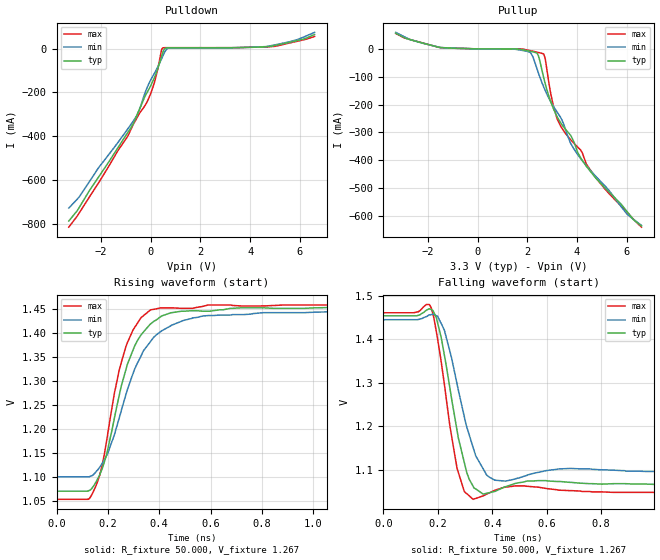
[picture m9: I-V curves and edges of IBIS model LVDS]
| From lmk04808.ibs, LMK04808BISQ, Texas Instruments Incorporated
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|   Model LVDS
[Model]   LVDS
Model_type   Output
Polarity   Non-Inverting
Vmeas = 1.25
Vref = 1.25
Cref = 0pF
Rref = 50
|   typ   min   max
|   (nom PVT)   (slow PVT)   (fast PVT)
C_comp   1.2694p   1.2464p   1.3920p
|C_comp (High state)   1.2694p   1.2464p   1.3920p
|C_comp (Low state)   1.7368p   1.7367p   1.7369p
[Voltage Range]   3.3   3.135   3.465
[Temperature Range]   45   125   -40
[Pullup Reference]   3.3   3.135   3.465
[Pulldown Reference]   0   0   0
[Power Clamp Reference]   3.3   3.135   3.465
[GND Clamp Reference]   0   0   0
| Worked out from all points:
|   slope of the pulldown table from 0 to 0.495 V, typ, clamps not added: 3.2 ohm
|   slope of the pullup table from 0 to 0.495 V, typ, clamps not added: 2.77 kohm
|   falling waveform, R_fixture 50.000, V_fixture 1.267: 20-80 % time 65.4ps typ, 78ps min, 57.7ps max; typ from 1.45 V to 1.07 V
|   rising waveform, R_fixture 50.000, V_fixture 1.267: 20-80 % time 113ps typ, 145ps min, 93.3ps max; typ from 1.07 V to 1.45 V
[Pulldown]
|   Voltage   I(typ)   I(min)   I(max)
-3.3V     -787.7mA   -728.5mA   -815.8mA
-2.869V   -723.8mA   -675.6mA   -748.8mA
-2.087V   -584.3mA   -542.1mA   -610.8mA
-686.4mV  -339.2mA   -328.2mA   -342.8mA
-468.6mV  -280.5mA   -281.5mA   -298.2mA
-181.5mV  -206.8mA   -187.5mA   -250.5mA
145.2mV   -132.5mA   -113mA     -154.9mA
476.8mV   -19.91mA   -35.88mA   2.577mA
561mV     564.3uA    -15.24mA   4.215mA
699.6mV   3.868mA    2.101mA    4.258mA
4.635V    8.376mA    9.221mA    7.753mA
6.595V    64.54mA    74.45mA    55.51mA
[Pullup]
|   Voltage   I(typ)   I(min)   I(max)
-3.3V     56.64mA    59.79mA    55.64mA
-1.488V   4.87mA     5.063mA    4.727mA
2.086V    -8.017mA   -10.91mA   -5.469mA
2.442V    -23.36mA   -85.47mA   -12.67mA
2.655V    -101.9mA   -135.9mA   -18.19mA
3.056V    -215.8mA   -207.2mA   -207mA
3.333V    -264.3mA   -245.2mA   -276.1mA
3.739V    -310mA     -338.7mA   -326.1mA
4.125V    -388.1mA   -391.9mA   -361.5mA
4.783V    -466.9mA   -460.8mA   -466.5mA
6.021V    -585.4mA   -594.9mA   -587.7mA
6.595V    -636.8mA   -634.7mA   -640.9mA
[Ramp]
R_load = 50
|   typ   min   max
dV/dt_r   0.231387/1.13087e-10   0.206921/1.44841e-10   0.243676/9.35061e-11
dV/dt_f   0.233919/6.51324e-11   0.206921/7.82597e-11   0.245855/5.7768e-11
[Falling Waveform]
R_fixture = 50.000
V_fixture = 1.267
V_fixture_min = 1.267
V_fixture_max = 1.267
C_fixture = 0.000
|  time   V(typ)   V(min)   V(max)
0s        1.454V     1.445V     1.461V
176.5ps   1.468V     1.457V     1.471V
194.9ps   1.449V     1.454V     1.416V
223.9ps   1.364V     1.421V     1.297V
270.7ps   1.19V      1.297V     1.103V
329.6ps   1.062V     1.151V     1.032V
379.2ps   1.046V     1.088V     1.044V
446.5ps   1.061V     1.074V     1.06V
685.4ps   1.071V     1.103V     1.052V
2ns       1.07V      1.1V       1.052V
[Rising Waveform]
R_fixture = 50.000
V_fixture = 1.267
V_fixture_min = 1.267
V_fixture_max = 1.267
C_fixture = 0.000
|  time   V(typ)   V(min)   V(max)
0s        1.07V      1.1V       1.053V
141.6ps   1.079V     1.104V     1.067V
168.1ps   1.104V     1.12V      1.103V
194.9ps   1.146V     1.144V     1.174V
225.6ps   1.223V     1.188V     1.275V
270.7ps   1.324V     1.272V     1.372V
315.3ps   1.384V     1.337V     1.42V
366.5ps   1.419V     1.382V     1.448V
590.9ps   1.445V     1.436V     1.458V
2ns       1.454V     1.445V     1.459V
